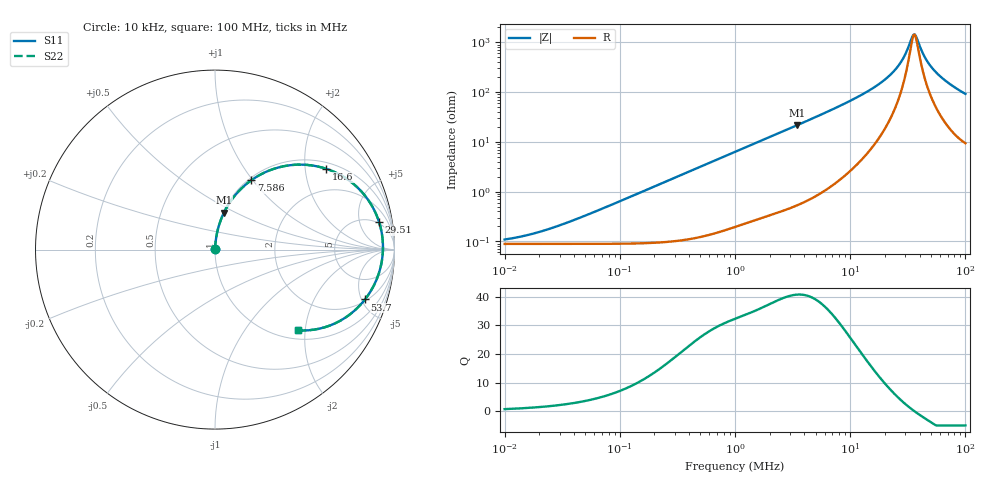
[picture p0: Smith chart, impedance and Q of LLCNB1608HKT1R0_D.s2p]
! LLCNB1608HKT1R0_D  S-PARAMETER MODEL  ( Standard Model )
! Model Generated by TAIYO YUDEN Corporation (http://www.ty-top.com)
! Version 1.0
! TAIYO YUDEN Control No. 200410
! Copyright(c) 2020 TAIYO YUDEN CO.,LTD. All Rights Reserved.
! Product Description (link to TY-COMPAS)
! https://ds.yuden.co.jp/TYCOMPAS/or/detail?pn=LLCNB1608HKT1R0MD&u=M
! Products Name : Inductors
! Characteristics :
!  Inductance : 1.0 [uH] , SRF(min) : - [Hz] , DC Resistance(max) : 110 [mOhm]
!  Rated Current : Saturation  2.2 [A] (dL = 30 [%]), Temp Rise  1.6 [A] (dT = 40 [degC])
!  Case Size : 1.6 x 0.8 / 0.063 x 0.031 [mm/inch] , Thickness : 0.8 / 0.031 [mm/inch]
!  (Conditions: Temperature = 25 [degC] , DC Bias Current = 0 [A])
! External Node Assignments :
!  1  o---GGG---o  2
! GND o---------o GND
! Frequency Range : 10kHz  -  100MHz  [ 402 STEP ]
# MHz S RI R 50
! Freq[MHz].  S11 Real  S11 Imag  S21 Real  S21 Imag  S12 Real  S12 Imag  S22 Real  S22 Imag
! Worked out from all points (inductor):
!   401 points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, 10 kHz to 100 MHz, reference 50 ohm
!   read as one part in series: L = 1.01 uH near 42.66 kHz
!   highest Q = 40.7 at 3.467 MHz (marker M1), where L = 995 nH
!   self-resonance near 36.05 MHz
!   S11 on the Smith chart (normalised r, x): 10 kHz: 1.00, +0.00; 7.586 MHz: 1.03, +0.98; 16.6 MHz: 1.19, +2.60; 29.51 MHz: 5, +10; 53.7 MHz: 2.15, -5.33; 100 MHz: 1.19, -1.83
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0.01  0.00089 0.000633  0.9991 -0.000633  0.9991 -0.000633  0.00089 0.000633
0.019953  0.000891 0.00126  0.9991 -0.00126  0.9991 -0.00126  0.000891 0.00126
0.046774  0.000899 0.00296  0.9991 -0.00296  0.9991 -0.00296  0.000899 0.00296
0.218776  0.00114 0.0139  0.9989 -0.0139  0.9989 -0.0139  0.00114 0.0139
1  0.00587 0.0624  0.9941 -0.0624  0.9941 -0.0624  0.00587 0.0624
1.949845  0.0177 0.1193  0.9823 -0.1193  0.9823 -0.1193  0.0177 0.1193
3.467369  0.0495 0.205  0.9505 -0.205  0.9505 -0.205  0.0495 0.205
4.677351  0.0854 0.2671  0.9146 -0.2671  0.9146 -0.2671  0.0854 0.2671
7.585776  0.2014 0.3858  0.7986 -0.3858  0.7986 -0.3858  0.2014 0.3858
12.02264  0.4157 0.4698  0.5843 -0.4698  0.5843 -0.4698  0.4157 0.4698
16.59587  0.6211 0.4499  0.3789 -0.4499  0.3789 -0.4499  0.6211 0.4499
21.87762  0.7928 0.347  0.2072 -0.347  0.2072 -0.347  0.7928 0.347
25.70396  0.8701 0.2508  0.1299 -0.2508  0.1299 -0.2508  0.8701 0.2508
29.51209  0.9142 0.1531  0.0858 -0.1531  0.0858 -0.1531  0.9142 0.1531
34.67368  0.9355 0.0301  0.0645 -0.0301  0.0645 -0.0301  0.9355 0.0301
36.30781  0.9355 -0.0054  0.0645 0.0054  0.0645 0.0054  0.9355 -0.0054
38.01894  0.9327 -0.0406  0.0673 0.0406  0.0673 0.0406  0.9327 -0.0406
44.66836  0.9033 -0.159  0.0967 0.159  0.0967 0.159  0.9033 -0.159
48.97788  0.8736 -0.2211  0.1264 0.2211  0.1264 0.2211  0.8736 -0.2211
53.70318  0.8358 -0.2778  0.1642 0.2778  0.1642 0.2778  0.8358 -0.2778
70.79458  0.6833 -0.404  0.3167 0.404  0.3167 0.404  0.6833 -0.404
100  0.4632 -0.4499  0.5368 0.4499  0.5368 0.4499  0.4632 -0.4499
